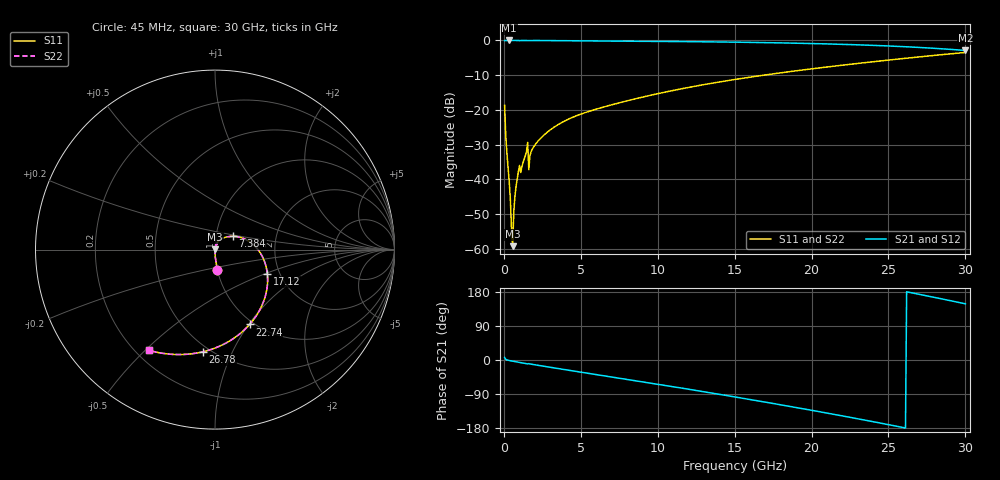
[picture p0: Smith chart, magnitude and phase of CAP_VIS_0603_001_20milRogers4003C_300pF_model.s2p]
! S-parameter model data by Modelithics Inc.  support@modelithics.com  813-866-6335  Tampa FL USA
! S-Parameter data specifications:
! Substrate: 20-mil Rogers 4003C, substrate thickness, H=0.508mm, Dielectric constant, Er=3.75
! PCB Mounting Pad Footprint: Pad width, PadW=0.90mm , Pad length, PadL=1.00mm , Pad gap, PadG (edge-to-edge)=1.00mm , Reference planes=3.0mm apart
! Created Wed Nov 18 13:33:45 2015
# hz S ma R 50
! 2 Port Network Data from SP1.SP block
! freq  magS11  angS11  magS21  angS21  magS12  angS12  magS22  angS22
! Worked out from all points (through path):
!   401 points, 45 MHz to 30 GHz, reference 50 ohm
!   highest |S21| = 0.00 dB at 344.6 MHz (marker M1); lowest = -2.9 dB at 30 GHz (marker M2)
!   group delay of S21, straight-line fit = 19.4 ps
!   lowest |S11| = -59.3 dB at 569.2 MHz (marker M3), VSWR 1.00, Z = 50.1 + j0.092 ohm
!   |S11| at or under -10 dB: start of sweep to 16.89 GHz
!   |S22| runs from -59.3 to -3.5 dB; largest |S21 - S12| = 0
!   S11 on the Smith chart (normalised r, x): 45 MHz: 1.00, -0.23; 7.384 GHz: 1.21, +0.18; 17.12 GHz: 1.72, -0.52; 22.74 GHz: 0.96, -1.01; 26.78 GHz: 0.46, -0.78; 30 GHz: 0.25, -0.51
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4.5e7  0.116 -83.5  0.9931 6.4  0.9931 6.4  0.116 -83.5
1.94775e8  0.0237 -88.9  0.9994 0.3  0.9994 0.3  0.0237 -88.9
3.4455e8  0.009222 -88.7  0.9995 -1.3  0.9995 -1.3  0.009222 -88.7
4.194375e8  0.00514 -86.8  0.9995 -2.0  0.9995 -2.0  0.00514 -86.8
4.94325e8  0.001909 -77.5  0.9995 -2.6  0.9995 -2.6  0.001909 -77.5
5.692125e8  0.001089 57.5  0.9994 -3.1  0.9994 -3.1  0.001089 57.5
6.441e8  0.003491 76.9  0.9994 -3.7  0.9994 -3.7  0.003491 76.9
8.687625e8  0.01032 80.2  0.9991 -5.3  0.9991 -5.3  0.01032 80.2
1.392975e9  0.02192 78.3  0.9986 -8.8  0.9986 -8.8  0.02192 78.3
1.767412e9  0.02495 76.3  0.9984 -11.0  0.9984 -11.0  0.02495 76.3
2.14185e9  0.03397 74.1  0.9978 -13.6  0.9978 -13.6  0.03397 74.1
3.115388e9  0.05352 66.7  0.9952 -19.9  0.9952 -19.9  0.05352 66.7
5.062462e9  0.08794 50.8  0.9853 -32.4  0.9853 -32.4  0.08794 50.8
7.383975e9  0.1245 36.3  0.9773 -47.0  0.9773 -47.0  0.1245 36.3
1.007992e10  0.1726 20.6  0.9694 -64.4  0.9694 -64.4  0.1726 20.6
1.50225e10  0.2743 -10.7  0.945 -97.5  0.945 -97.5  0.2743 -10.7
1.711935e10  0.3214 -24.8  0.9297 -112.0  0.9297 -112.0  0.3214 -24.8
2.003996e10  0.3907 -45.3  0.9023 -132.9  0.9023 -132.9  0.3907 -45.3
2.273591e10  0.4594 -65.2  0.8688 -153.0  0.8688 -153.0  0.4594 -65.2
2.505742e10  0.5231 -83.0  0.8316 -171.0  0.8316 -171.0  0.5231 -83.0
2.677984e10  0.5732 -96.7  0.7978 175.1  0.7978 175.1  0.5732 -96.7
3e10  0.6716 -123.4  0.7172 148.3  0.7172 148.3  0.6716 -123.4
